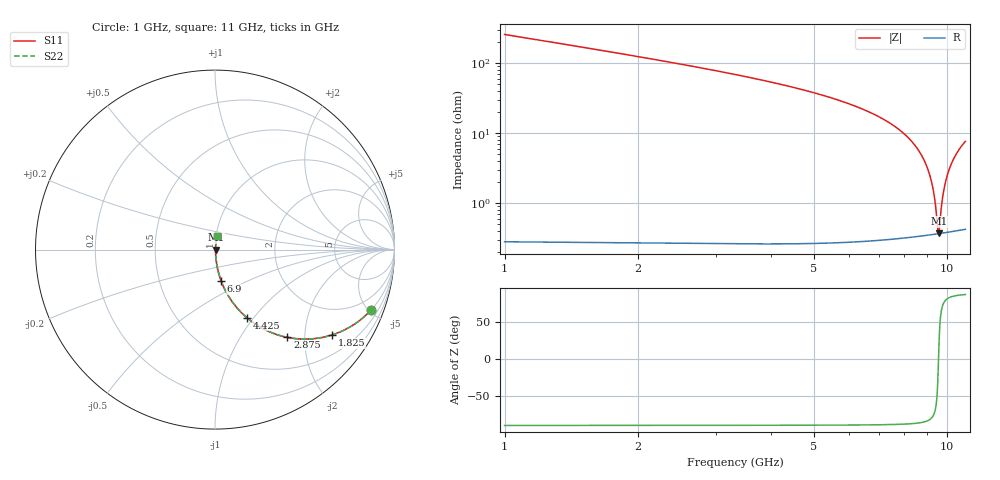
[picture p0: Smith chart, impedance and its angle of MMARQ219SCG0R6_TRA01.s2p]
! MMARQ219SCG0R6_TRA01  S-PARAMETER MODEL  ( General Type )
! Model Generated by TAIYO YUDEN Corporation (http://www.ty-top.com)
! Version 1.0
! TAIYO YUDEN Control No. 160201
! Copyright(c) 2016 TAIYO YUDEN CO.,LTD. All Rights Reserved.
! Product Description (link to TY-COMPAS)
! https://ds.yuden.co.jp/TYCOMPAS/or/detail?pn=MMARQ219SCG0R6BTRA01&u=M
! Products Name : Multilayer Ceramic Capacitors
! Characteristics :
!  Capacitance : 0.6 pF , Rated Voltage : 250V , TCC : CG / C0G
!  Case Size : 2.0 x 1.25 / 0.079 x 0.049 [mm/inch] , Thickness : 0.85 / 0.033 [mm/inch]
!  (Conditions: Temperature = 25 degC , DC Bias Current/Voltage = 0A / 0V)
! External Node Assignments :
!  1  o---| |---o  2
! GND o---------o GND
! Frequency Range : 1000MHz  -  11000MHz  [ 401 STEP ]
# MHz S RI R 50
! Freq[MHz].  S11 Real  S11 Imag  S21 Real  S21 Imag  S12 Real  S12 Imag  S22 Real  S22 Imag
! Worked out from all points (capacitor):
!   401 points, 1 GHz to 11 GHz, reference 50 ohm
!   read as one part in series: C = 613 fF near 1.05 GHz
!   lowest |Z| = 370 mohm at 9.575 GHz (marker M1)
!   series resonance near 9.566 GHz, so ESL is about 450 pH
!   S11 on the Smith chart (normalised r, x): 1 GHz: 1.01, -5.14; 1.825 GHz: 1.01, -2.74; 2.875 GHz: 1.01, -1.64; 4.425 GHz: 1.01, -0.92; 6.9 GHz: 1.01, -0.36; 11 GHz: 1.01, +0.15
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1000  0.8681 -0.3379  0.1319 0.3379  0.1319 0.3379  0.8681 -0.3379
1825  0.6525 -0.4752  0.3475 0.4752  0.3475 0.4752  0.6525 -0.4752
2675  0.4449 -0.4955  0.5551 0.4955  0.5551 0.4955  0.4449 -0.4955
2875  0.4034 -0.489  0.5966 0.489  0.5966 0.489  0.4034 -0.489
4350  0.1847 -0.3853  0.8153 0.3853  0.8153 0.3853  0.1847 -0.3853
4425  0.177 -0.3788  0.823 0.3788  0.823 0.3788  0.177 -0.3788
6000  0.0668 -0.2445  0.9332 0.2445  0.9332 0.2445  0.0668 -0.2445
6900  0.0343 -0.174  0.9657 0.174  0.9657 0.174  0.0343 -0.174
7675  0.0173 -0.1182  0.9827 0.1182  0.9827 0.1182  0.0173 -0.1182
8325  0.0089 -0.0748  0.9911 0.0748  0.9911 0.0748  0.0089 -0.0748
8800  0.00543 -0.045  0.9946 0.045  0.9946 0.045  0.00543 -0.045
9125  0.00415 -0.0254  0.9959 0.0254  0.9959 0.0254  0.00415 -0.0254
9350  0.00373 -0.0123  0.9963 0.0123  0.9963 0.0123  0.00373 -0.0123
9525  0.00364 -0.00229  0.9964 0.00229  0.9964 0.00229  0.00364 -0.00229
9575  0.00365 0.000531  0.9963 -0.000531  0.9963 -0.000531  0.00365 0.000531
9625  0.00368 0.00334  0.9963 -0.00334  0.9963 -0.00334  0.00368 0.00334
9725  0.00379 0.00892  0.9962 -0.00892  0.9962 -0.00892  0.00379 0.00892
9800  0.0039 0.0131  0.9961 -0.0131  0.9961 -0.0131  0.0039 0.0131
9900  0.00412 0.0185  0.9959 -0.0185  0.9959 -0.0185  0.00412 0.0185
10050  0.00454 0.0266  0.9955 -0.0266  0.9955 -0.0266  0.00454 0.0266
10450  0.00627 0.0476  0.9937 -0.0476  0.9937 -0.0476  0.00627 0.0476
11000  0.00991 0.0751  0.9901 -0.0751  0.9901 -0.0751  0.00991 0.0751
